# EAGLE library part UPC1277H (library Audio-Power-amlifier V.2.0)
The uPC1277H is a dual audio power ampliifier designed for a stereo radio cassette and in a 12-pin SIP power single in line plastic package.The uPC1277H has two audio power amplifiers and each of two provides 4,2 W output power at 12V/4 OHMS.
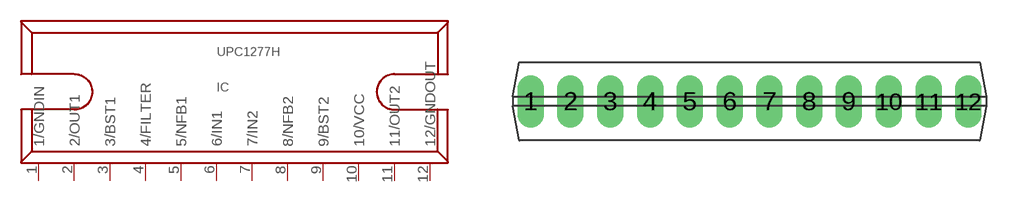
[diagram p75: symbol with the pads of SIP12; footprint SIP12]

Designator prefix IC

## UPC1277H  [SIP12]
1  1/GNDIN  pwr
2  2/OUT1  out
3  3/BST1
4  4/FILTER
5  5/NFB1
6  6/IN1  in
7  7/IN2  in
8  8/NFB2
9  9/BST2
10  10/VCC  pwr
11  11/OUT2  out
12  12/GNDOUT  pwr

## Footprint SIP12 (pad centres in mm)
drill 0.8 pad 1.676 long: 1 -13.97,0; 2 -11.43,0; 3 -8.89,0; 4 -6.35,0; 5 -3.81,0; 6 -1.27,0; 7 1.27,0; 8 3.81,0; 9 6.35,0; 10 8.89,0; 11 11.43,0; 12 13.97,0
